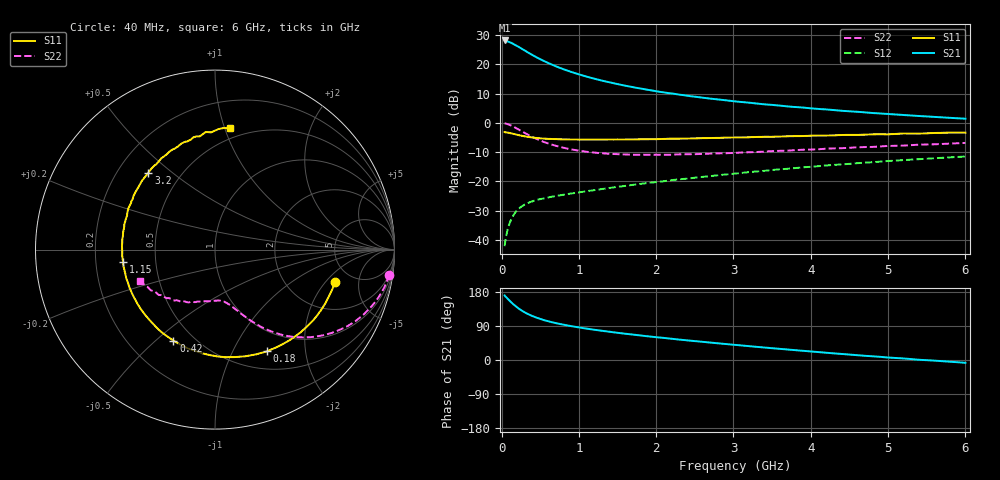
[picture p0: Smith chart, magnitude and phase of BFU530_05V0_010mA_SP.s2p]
! Filename:  P:\Prog\Test\Noise\ATS_data\Testdata_Net\03 Spar\BFU530_APG2013_40_A05_05p0V_010mA_SP_CM01_D.s2p
! Date/Time: Fri 26/Apr/2013 13:03:15
! BFU530_APG2013_40_A05_05p0V_1to25mA_SP_CM01_Bias5_R.s2p
! MDIF S-parameter v. bias file
! BFU530_APG2013_40_A05_05p0V_1to25mA_SP_CM01
! Date/time Wed Apr 24 19:36:53 2013
! VAR V_out= 5.0000
! VAR I_out= 10.0050
! VAR V_in= 0.8308
! VAR I_in= 0.1098
! Device data file deembeded for feedlines and parallel
! Original file: \03 Spar\BFU530_APG2013_40_A05_05p0V_010mA_SP_CM01_R.s2p
! Feed-files: PR047V01_250413_Feed1.s2p, PR047V01_250413_Feed2.s2p
! Parallel-file: PR047V01_250413_Par.s2p
# MHz S MA R 50
!  Freq-MHz  S11-mag  S11-arg  S21-mag  S21-arg  S12-mag  S12-arg  S22-mag  S22-arg
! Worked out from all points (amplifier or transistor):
!   98 points, 40 MHz to 6 GHz, reference 50 ohm
!   highest |S21| = 28.2 dB at 40 MHz (marker M1)
!   |S21| within 3 dB of that: start of sweep to 271.6 MHz
!   unconditionally stable (mu >= 1): 1.721 GHz to 3.894 GHz
!   at 300 MHz: K = 0.31, MSG = 26.4 dB, |S12| = -28.0 dB
!   at 1.6 GHz: K = 0.98, MSG = 17.1 dB, |S12| = -21.6 dB
!   at 6 GHz: K = 0.87, MSG = 6.5 dB, |S12| = -11.5 dB
!   S11 on the Smith chart (normalised r, x): 40 MHz: 3.65, -2.56; 180 MHz: 0.72, -1.37; 420 MHz: 0.39, -0.57; 1.15 GHz: 0.32, -0.06; 3.2 GHz: 0.33, +0.42; 6 GHz: 0.42, +1.04
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40  0.6939 -15.2  25.66 170.4  0.007773 82.9  0.9797 -8.2
50  0.6895 -19.0  25.59 167.5  0.009666 81.3  0.9739 -10.3
120  0.6636 -44.0  23.55 153.2  0.02152 70.2  0.9036 -23.6
140  0.6542 -50.6  22.86 149.4  0.02443 67.5  0.8781 -27.0
180  0.6365 -62.9  21.37 142.5  0.02953 62.5  0.8241 -33.0
220  0.6178 -74.2  20 136.2  0.0337 58.6  0.7704 -38.2
300  0.5879 -93.2  17.28 125.8  0.04004 52.7  0.6722 -46.6
360  0.5714 -104.9  15.5 119.6  0.04357 49.7  0.6106 -51.4
420  0.5574 -114.6  13.97 114.3  0.04643 47.7  0.5571 -55.2
480  0.548 -123.0  12.67 109.9  0.04888 46.2  0.5133 -58.3
550  0.5371 -131.7  11.4 105.2  0.05104 45.2  0.469 -61.3
650  0.5298 -141.4  9.932 99.9  0.05448 44.4  0.4249 -64.8
800  0.5226 -152.9  8.28 93.2  0.05892 44.5  0.3757 -68.7
1050  0.5174 -167.7  6.46 84.3  0.06614 45.5  0.3273 -74.0
1150  0.5169 -172.3  5.929 81.3  0.06917 46.0  0.3147 -75.7
1600  0.5197 170.4  4.319 69.3  0.08346 47.9  0.2878 -83.6
2050  0.5285 157.8  3.391 59.2  0.09865 48.8  0.2845 -91.4
3100  0.5636 132.5  2.274 38.4  0.1389 47.7  0.3107 -110.0
3200  0.5669 130.9  2.214 36.6  0.1437 47.4  0.3142 -111.3
4100  0.6056 112.9  1.728 20.9  0.1814 42.9  0.3532 -127.0
5200  0.6569 94.5  1.362 4.1  0.2306 35.3  0.4081 -145.0
6000  0.6799 82.9  1.177 -7.4  0.2653 28.4  0.4537 -157.5
